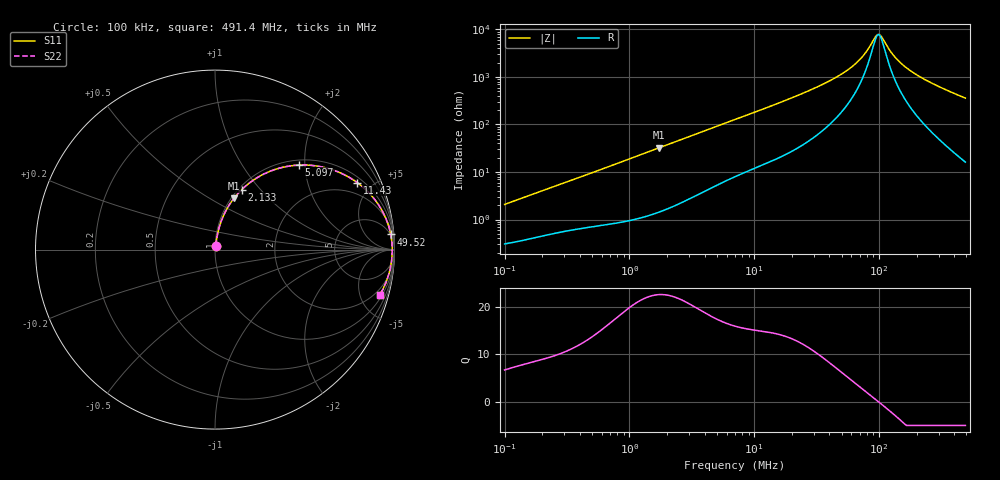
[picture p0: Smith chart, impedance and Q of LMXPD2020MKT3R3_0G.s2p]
! LMXPD2020MKT3R3_0G  S-PARAMETER MODEL  ( General Type )
! Model Generated by TAIYO YUDEN Corporation (http://www.ty-top.com)
! Version 1.0
! TAIYO YUDEN Control No. 191023NI43SB-FBB
! Copyright(c) 2019 TAIYO YUDEN CO.,LTD. All Rights Reserved.
! Product Description (link to TY-COMPAS)
! https://ds.yuden.co.jp/TYCOMPAS/or/detail?pn=LMXPD2020MKT3R3M0G&u=M
! Products Name : Inductors
! Characteristics :
!  Inductance : 3.3 uH , SRF(min) : -Hz , DC Resistance(max) : 0.2724 Ohm
!  Rated Current : Saturation :1250 mA , Temp Rise : 900 mA
!  Case Size : 2.0 x 2.0 / 0.079 x 0.079 [mm/inch] , Thickness : 1.2 / 0.047 [mm/inch]
!  (Conditions: Temperature = 25 degC , DC Bias Current/Voltage = 0A / 0V)
! External Node Assignments :
!  1  o---GGG---o  2
! GND o---------o GND
! Frequency Range : 0.1MHz  -  491.415554MHz  [ 402 STEP ]
# MHz S RI R 50
! Freq[MHz].  S11 Real  S11 Imag  S21 Real  S21 Imag  S12 Real  S12 Imag  S22 Real  S22 Imag
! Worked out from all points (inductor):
!   401 points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, 100 kHz to 491.4 MHz, reference 50 ohm
!   read as one part in series: L = 3.25 uH near 104.3 kHz
!   highest Q = 22.6 at 1.724 MHz (marker M1), where L = 2.98 uH
!   self-resonance near 97.74 MHz
!   S11 on the Smith chart (normalised r, x): 100 kHz: 1.01, +0.04; 2.133 MHz: 1.04, +0.80; 5.097 MHz: 1.11, +1.87; 11.43 MHz: 1.27, +4.09; 49.52 MHz: 5, +22; 491.4 MHz: 1.32, -7.17
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0.1  0.00348 0.0205  0.9965 -0.0205  0.9965 -0.0205  0.00348 0.0205
0.415258  0.0127 0.0786  0.9873 -0.0786  0.9873 -0.0786  0.0127 0.0786
0.873614  0.0346 0.158  0.9654 -0.158  0.9654 -0.158  0.0346 0.158
1.72439  0.1049 0.2852  0.8951 -0.2852  0.8951 -0.2852  0.1049 0.2852
2.13266  0.1481 0.3336  0.8519 -0.3336  0.8519 -0.3336  0.1481 0.3336
3.193489  0.2703 0.4201  0.7297 -0.4201  0.7297 -0.4201  0.2703 0.4201
5.096771  0.4684 0.471  0.5316 -0.471  0.5316 -0.471  0.4684 0.471
7.010104  0.6116 0.457  0.3884 -0.457  0.3884 -0.457  0.6116 0.457
11.42833  0.7927 0.3732  0.2073 -0.3732  0.2073 -0.3732  0.7927 0.3732
17.48055  0.8925 0.2757  0.1075 -0.2757  0.1075 -0.2757  0.8925 0.2757
29.11  0.9537 0.1692  0.0463 -0.1692  0.0463 -0.1692  0.9537 0.1692
49.51738  0.9791 0.0843  0.0209 -0.0843  0.0209 -0.0843  0.9791 0.0843
71.06312  0.9856 0.0382  0.0144 -0.0382  0.0144 -0.0382  0.9856 0.0382
79.02916  0.9866 0.0257  0.0134 -0.0257  0.0134 -0.0257  0.9866 0.0257
93.67342  0.9874 0.00619  0.0126 -0.00619  0.0126 -0.00619  0.9874 0.00619
97.74029  0.9874 0.00135  0.0126 -0.00135  0.0126 -0.00135  0.9874 0.00135
104.174  0.9874 -0.00591  0.0126 0.00591  0.0126 0.00591  0.9874 -0.00591
120.8815  0.987 -0.023  0.013 0.023  0.013 0.023  0.987 -0.023
149.5017  0.9853 -0.0483  0.0147 0.0483  0.0147 0.0483  0.9853 -0.0483
197.0689  0.9804 -0.0843  0.0196 0.0843  0.0196 0.0843  0.9804 -0.0843
295.0951  0.9652 -0.1475  0.0348 0.1475  0.0348 0.1475  0.9652 -0.1475
491.4156  0.9182 -0.2525  0.0818 0.2525  0.0818 0.2525  0.9182 -0.2525
